FUNCTION_BLOCK PS_UnitModeManager
VAR_INPUT
	Execute 		: BOOL;
	eModeCommand 	: E_PMLUnitMode;
	ePMLState		: E_PMLState;
END_VAR
VAR_OUTPUT
	eModeStatus 	: E_PMLUnitMode;
	Done 			: BOOL;
	Error 			: BOOL;
	ErrorID 		: UDINT;
END_VAR
VAR
	rTrig			: R_TRIG;
END_VAR

rTrig(CLK:= Execute);

IF rTrig.Q THEN (* rising edge Execute *)
	Done := FALSE;
	Error := FALSE;
	ErrorID := 0;

     CASE eModeStatus OF
           ePMLUnitMode_UNDEFINED:
                eModeStatus := eModeCommand;
                Done := TRUE;

		ePMLUnitMode_AUTOMATIC:
			IF (ePMLState = ePMLState_STOPPED) OR (ePMLState = ePMLState_ABORTED) OR (ePMLState = ePMLState_IDLE) THEN
				eModeStatus := eModeCommand;
				Done := TRUE;
			ELSIF ((ePMLState = ePMLState_SUSPENDED) OR (ePMLState = ePMLState_HELD) OR (ePMLState = ePMLState_COMPLETE))
				AND (eModeCommand = ePMLUnitMode_SEMIAUTOMATIC) THEN

				eModeStatus := eModeCommand;
				Done := TRUE;
			ELSIF (ePMLState = ePMLState_HELD) AND (eModeCommand = ePMLUnitMode_MAINTENANCE) THEN
				eModeStatus := eModeCommand;
				Done := TRUE;
			ELSE
				Error := TRUE;
				ErrorID := 1;
			END_IF

		ePMLUnitMode_MAINTENANCE:
			IF (ePMLState = ePMLState_STOPPED) OR (ePMLState = ePMLState_ABORTED) OR (ePMLState = ePMLState_IDLE) THEN
				eModeStatus := eModeCommand;
				Done := TRUE;
			ELSIF (ePMLState = ePMLState_HELD) AND ((eModeCommand = ePMLUnitMode_AUTOMATIC) OR (eModeCommand = ePMLUnitMode_SEMIAUTOMATIC)) THEN
				eModeStatus := eModeCommand;
				Done := TRUE;
			ELSE
				Error := TRUE;
				ErrorID := 1;
			END_IF

		ePMLUnitMode_MANUAL:
			IF (ePMLState = ePMLState_STOPPED) OR (ePMLState = ePMLState_ABORTED) OR (ePMLState = ePMLState_IDLE) THEN
				eModeStatus := eModeCommand;
				Done := TRUE;
			ELSE
				Error := TRUE;
				ErrorID := 1;
			END_IF

		ePMLUnitMode_SEMIAUTOMATIC:
			IF (ePMLState = ePMLState_STOPPED) OR (ePMLState = ePMLState_ABORTED) OR (ePMLState = ePMLState_IDLE) THEN
				eModeStatus := eModeCommand;
				Done := TRUE;
			ELSIF ((ePMLState = ePMLState_SUSPENDED) OR (ePMLState = ePMLState_HELD) OR (ePMLState = ePMLState_COMPLETE))
				AND (eModeCommand = ePMLUnitMode_AUTOMATIC) THEN

				eModeStatus := eModeCommand;
				Done := TRUE;
			ELSIF (ePMLState = ePMLState_HELD) AND (eModeCommand = ePMLUnitMode_MAINTENANCE) THEN
				eModeStatus := eModeCommand;
				Done := TRUE;
			ELSE
				Error := TRUE;
				ErrorID := 1;
			END_IF

		ePMLUnitMode_DRYRUN:
			eModeStatus := eModeCommand;
			Done := TRUE;

		ePMLUnitMode_USERMODE1:
			eModeStatus := eModeCommand;
			Done := TRUE;

		ePMLUnitMode_USERMODE2:
			eModeStatus := eModeCommand;
			Done := TRUE;

		ePMLUnitMode_IDLE:
			IF (ePMLState = ePMLState_STOPPED) OR (ePMLState = ePMLState_ABORTED) OR (ePMLState = ePMLState_IDLE) THEN
				eModeStatus := eModeCommand;
				Done := TRUE;
			ELSE
				Error := TRUE;
				ErrorID := 1;
			END_IF

           ePMLUnitMode_ESTOP:
                IF (ePMLState = ePMLState_STOPPED) OR (ePMLState = ePMLState_ABORTED) OR (ePMLState = ePMLState_IDLE) THEN
                     eModeStatus := eModeCommand;
                     Done := TRUE;
                ELSE
                     Error := TRUE;
                     ErrorID := 1;
                END_IF
     END_CASE
END_IF

 (* reset with bExecute = FALSE *)
 IF NOT Execute THEN
     Done := FALSE;
     Error := FALSE;
     ErrorID := 0;
 END_IF

END_FUNCTION_BLOCK
